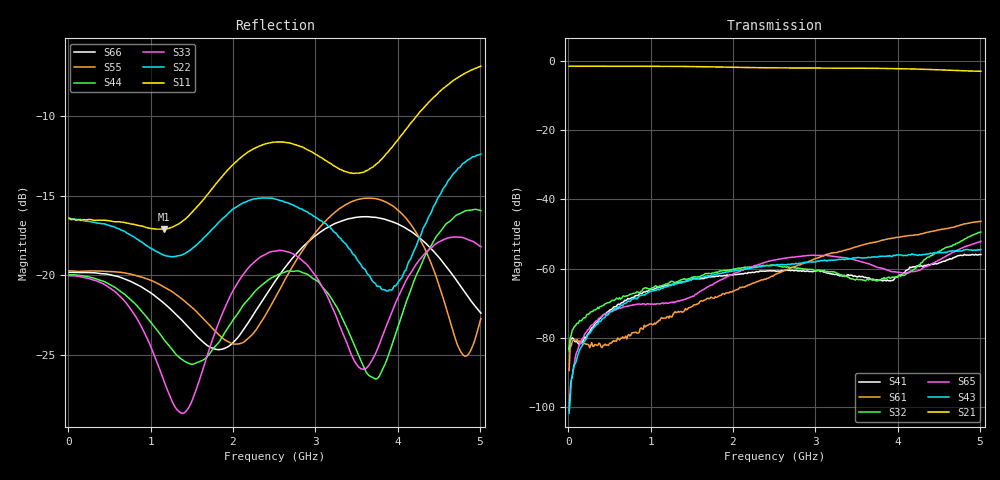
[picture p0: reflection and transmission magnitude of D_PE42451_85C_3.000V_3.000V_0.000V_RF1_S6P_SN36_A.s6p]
! Device ID: PE42451
! Serial: 36
! Insertion: A
! Temp: 85C
! VDD: 3.000
! Control_Hi: 100.000
! Control_Lo: 0.000
! Logic State: RF1
! Port 1: RFC
! Port 2: RF1
! Port 3: RF2
! Port 4: RF3
! Port 5: RF4
! Port 6: RF5
! V1 = 3.00
! V2 = 0.00
! V3 = 0.00
! V4 = 0.00
! IDD: 1.414240e-05
#  Hz  S  RI  R  50
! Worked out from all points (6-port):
!   401 points, 10 MHz to 5.01 GHz, reference 50 ohm
!   strongest paths, dB at 10 MHz, 1.26 GHz, 2.51 GHz, 3.76 GHz, 5.01 GHz:
!     S21: -1.6, -1.6, -2.0, -2.2, -3.0
!     S43: -101.8, -64.5, -59.1, -56.6, -54.5
!     S65: -101.0, -69.8, -57.5, -59.7, -52.2
!     S32: -83.8, -63.7, -59.1, -63.5, -49.5
!     S61: -89.5, -74.0, -61.8, -52.2, -46.4
!     S41: -83.2, -64.6, -60.7, -63.3, -55.9
!   lowest |S11| = -17.1 dB at 1.16 GHz (marker M1), VSWR 1.32, Z = 57.9 - j13 ohm
!   |S11| at or under -10 dB: start of sweep to 4.224 GHz
